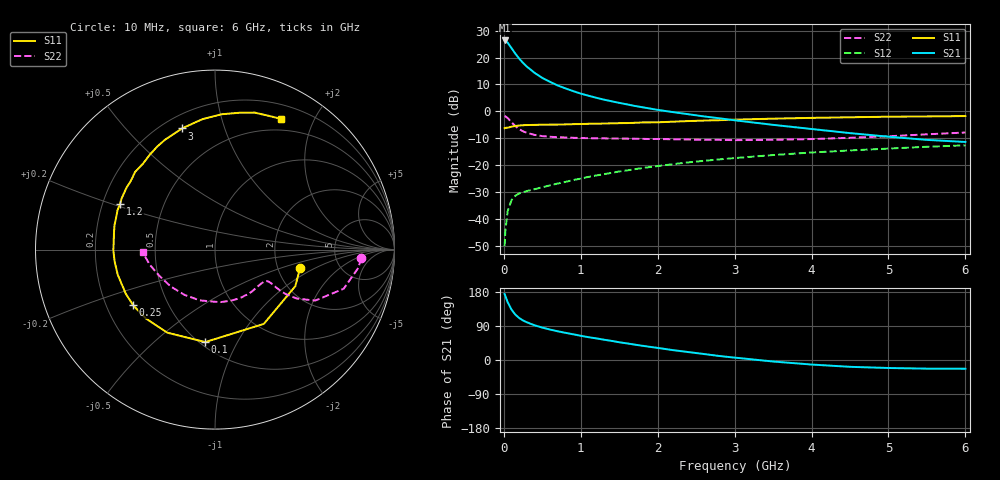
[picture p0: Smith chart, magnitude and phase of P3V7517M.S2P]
! SIEMENS Small Signal Semiconductors
! BFP181
! Si NPN RF Bipolar Junction Transistor in SOT143
! VCE = 0.75 V  IC = 17 mA
! Common Emitter S-Parameters:  March  1996
# GHz  S  MA  R  50
!  f  S11  S21  S12  S22
! GHz  MAG  ANG  MAG  ANG  MAG  ANG  MAG  ANG
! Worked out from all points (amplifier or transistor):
!   36 points, 10 MHz to 6 GHz, reference 50 ohm
!   highest |S21| = 26.4 dB at 10 MHz (marker M1)
!   |S21| within 3 dB of that: start of sweep to 102.9 MHz
!   unconditionally stable (mu >= 1): start of sweep to 22.83 MHz; 223.6 MHz to end of sweep
!   at 250 MHz: K = 1.09, MAG = 22.2 dB, |S12| = -30.1 dB
!   at 1.4 GHz: K = 2.50, MAG = 6.5 dB, |S12| = -22.9 dB
!   at 6 GHz: K = 2.35, MAG = -5.9 dB, |S12| = -12.7 dB
!   S11 on the Smith chart (normalised r, x): 10 MHz: 2.65, -0.73; 100 MHz: 0.53, -0.75; 250 MHz: 0.31, -0.28; 1.2 GHz: 0.27, +0.21; 3 GHz: 0.27, +0.73; 6 GHz: 0.36, +1.56
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0.01  0.485 -12.5  20.8 174.3  0.0031 72.8  0.816 -3.4
0.02  0.4917 -24.5  20.63 168.8  0.0061 75.8  0.8053 -7.2
0.05  0.4953 -56.7  18.91 152.6  0.0139 67.3  0.7496 -16.9
0.1  0.518 -96.0  14.93 132.8  0.0223 51.5  0.6261 -27.0
0.15  0.5338 -119.9  11.8 119.6  0.0269 44.6  0.5306 -30.9
0.2  0.544 -135.2  9.554 110.7  0.0297 41.4  0.4656 -32.2
0.25  0.5514 -145.8  7.943 104.2  0.0313 39.4  0.4242 -32.1
0.3  0.5545 -153.7  6.775 99.5  0.0329 39.3  0.3972 -31.7
0.4  0.5597 -165.5  5.194 91.5  0.0356 40.3  0.364 -30.9
0.5  0.5629 -173.1  4.179 85.5  0.0387 41.1  0.3457 -30.9
0.6  0.5664 -179.4  3.537 80.4  0.042 43.5  0.3364 -31.4
0.7  0.5665 174.8  3.025 75.8  0.0453 45.5  0.3296 -32.2
0.9  0.5764 166.2  2.38 67.9  0.0526 47.6  0.3218 -35.1
1.1  0.586 158.0  1.951 60.2  0.0603 49.1  0.3163 -38.8
1.2  0.5869 154.3  1.788 57.1  0.0639 49.6  0.3147 -40.8
1.7  0.6114 138.5  1.261 40.6  0.0837 49.6  0.3087 -52.1
2.2  0.6416 124.5  0.966 26.0  0.104 47.4  0.3018 -65.4
3  0.6997 105.2  0.681 6.3  0.135 41.5  0.2909 -89.7
3.5  0.7302 95.5  0.56 -4.0  0.1536 37.2  0.2953 -106.8
4.5  0.7744 79.9  0.393 -18.0  0.1872 27.6  0.3214 -140.5
5.5  0.8028 68.3  0.294 -22.8  0.2191 18.3  0.3733 -167.0
6  0.8155 63.3  0.269 -23.1  0.2329 13.2  0.4035 -178.0
